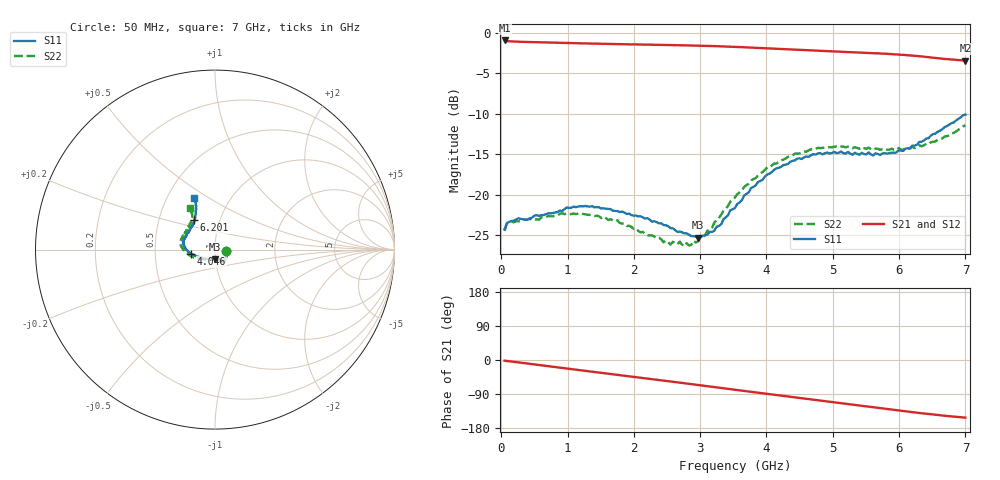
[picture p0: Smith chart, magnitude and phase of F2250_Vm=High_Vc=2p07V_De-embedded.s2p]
! Integrated Device Technology
! Corporate Headquarters
! 6024 Silver Creek Valley Road
! San Jose, CA 95138  USA
! Phone:  1-408-284-8200
! Toll Free:  1-800-223-1366
! Webpage:  http://www.idt.com/
! Timing and RF Division
! 515 Groton Road, Suite 102
! Westford, MA 01886-6024
! Device:  F2250
! Description: Voltage Variable RF Attenuator
! Frequency:  50.0 -  6000.00 MHz
! Package:  3x3 mm Thin QFN Plastic Package: 16 pin
! Ports:  2 RF, 3 DC
!  Pin  1  = GND
!  Pin  2  = NC
!  Pin  3  = RF1  = Port 1
!  Pin  4  = NC
!  Pin  5  = GND
!  Pin  6  = GND
!  Pin  7  = GND
!  Pin  8  = GND
!  Pin  9  = NC
!  Pin 10  = RF2  = Port 2
!  Pin 11  = NC
!  Pin 12  = GND
!  Pin 13  = GND
!  Pin 14  = VCNTRL
!  Pin 15  = VDD
!  Pin 16  = VMODE
! Vcntrl:  2.070 Volts
! Vmode:  +3.300 Volts
! Vdd:  +3.30  Volts
! Current:  1.319 mA
! Data:  The device was measured on a the F2250 evaluation board which has
!  individual transmission lines to the RF pins.  Data was collected
!  using a calibrated network analyzer.  The evaluation board was
!  de-embedded using a TRL calibration technique.
!  The reference plane is the edge of the package pin.
! Misc:  SN 10
!  Action Tracker AT0258
! Date Measured:  2014-11-26
! Date:  2015-10-15  MJV
! Note:
!  Integrated Device Technology supplies this data as a sample of measured
!  data at the package pin for this product.  Your particular data for this
!  product may vary.
!  Data was taken at 25 degrees C.
!  Integrated Device Technology reserves the right to change this data at anytime.
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# GHz S dB R 50
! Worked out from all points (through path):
!   201 points, 50 MHz to 7 GHz, reference 50 ohm
!   highest |S21| = -0.98 dB at 50 MHz (marker M1); lowest = -3.5 dB at 7 GHz (marker M2)
!   group delay of S21, straight-line fit = 61.1 ps
!   lowest |S11| = -25.3 dB at 2.969 GHz (marker M3), VSWR 1.11, Z = 49.7 - j5.4 ohm
!   |S11| at or under -10 dB: start of sweep to end of sweep
!   |S22| runs from -26.4 to -11.4 dB; largest |S21 - S12| = 0.0019
!   S11 on the Smith chart (normalised r, x): 50 MHz: 1.13, -0.02; 4.046 GHz: 0.76, -0.04; 6.201 GHz: 0.75, +0.26; 7 GHz: 0.68, +0.43
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0.05  -24.27 -9.2  -0.98 -1.8  -0.98 -1.8  -24.47 -9.7
0.08475  -23.49 -8.4  -1.05 -2.5  -1.05 -2.5  -23.57 -8.7
0.1195  -23.38 -9.0  -1.08 -3.3  -1.08 -3.2  -23.38 -8.2
0.91875  -22.01 -45.8  -1.27 -21.0  -1.27 -21.1  -22.28 -48.4
1.2315  -21.45 -53.5  -1.34 -27.9  -1.34 -27.9  -22.39 -58.9
1.75275  -22.03 -60.4  -1.43 -39.1  -1.43 -39.1  -23.18 -66.4
2.37825  -23.54 -60.8  -1.52 -52.7  -1.52 -52.8  -25.32 -69.0
2.552  -24.13 -65.2  -1.54 -56.6  -1.54 -56.6  -26.17 -75.6
2.691  -24.55 -72.1  -1.57 -59.7  -1.57 -59.7  -25.79 -82.6
2.7605  -24.78 -74.1  -1.58 -61.3  -1.58 -61.3  -26.36 -87.0
2.969  -25.33 -89.8  -1.62 -65.9  -1.62 -66.0  -25.76 -104.4
3.21225  -24.46 -118.8  -1.68 -71.4  -1.68 -71.5  -23.47 -128.0
3.525  -21.64 -146.0  -1.77 -78.5  -1.77 -78.5  -20.36 -146.7
3.76825  -19.18 -159.9  -1.86 -84.0  -1.87 -84.0  -18.26 -158.0
4.04625  -17.41 -170.2  -1.97 -90.2  -1.98 -90.2  -16.61 -168.6
4.4285  -15.78 179.1  -2.12 -98.6  -2.13 -98.6  -14.94 179.8
4.7065  -15.00 171.9  -2.22 -104.8  -2.22 -104.8  -14.45 173.9
5.054  -14.86 163.6  -2.35 -112.4  -2.35 -112.5  -14.06 166.7
5.85325  -14.90 137.4  -2.65 -129.9  -2.65 -130.1  -14.47 147.7
6.20075  -13.94 125.4  -2.86 -137.7  -2.86 -137.7  -14.07 138.6
6.54825  -12.47 117.1  -3.13 -144.7  -3.13 -144.8  -13.43 127.2
7  -10.12 111.9  -3.45 -152.0  -3.46 -152.1  -11.44 120.9
